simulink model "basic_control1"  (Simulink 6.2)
settings: Solver=ode45  StartTime=0.0  StopTime=10.0  RelTol=1e-3

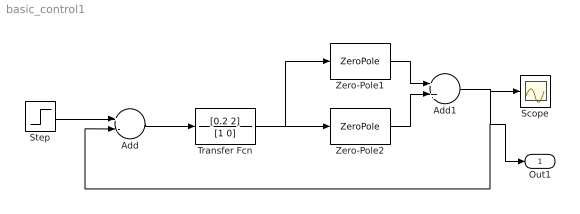
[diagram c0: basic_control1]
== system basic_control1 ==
  Add : Sum  Inputs=+-  OutScaling=2^-10
  Add1 : Sum  OutScaling=2^-10
  Scope : Scope
  Step : Step  Time=0  SampleTime=0
  Transfer Fcn : TransferFcn  Numerator=[0.2 2]  Denominator=[1 0]
  Zero-Pole1 : ZeroPole  Zeros=[]  Poles=[ -1]
  Zero-Pole2 : ZeroPole  Zeros=[ 0]  Poles=[-3 -4]  Gain=2
  Out1 : Outport
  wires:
  Add/1 -> Transfer Fcn/1
  Transfer Fcn/1 -> Zero-Pole1/1, Zero-Pole2/1
  Zero-Pole1/1 -> Add1/1
  Zero-Pole2/1 -> Add1/2
  Add1/1 -> Scope/1, Add/2, Out1/1
  Step/1 -> Add/1
